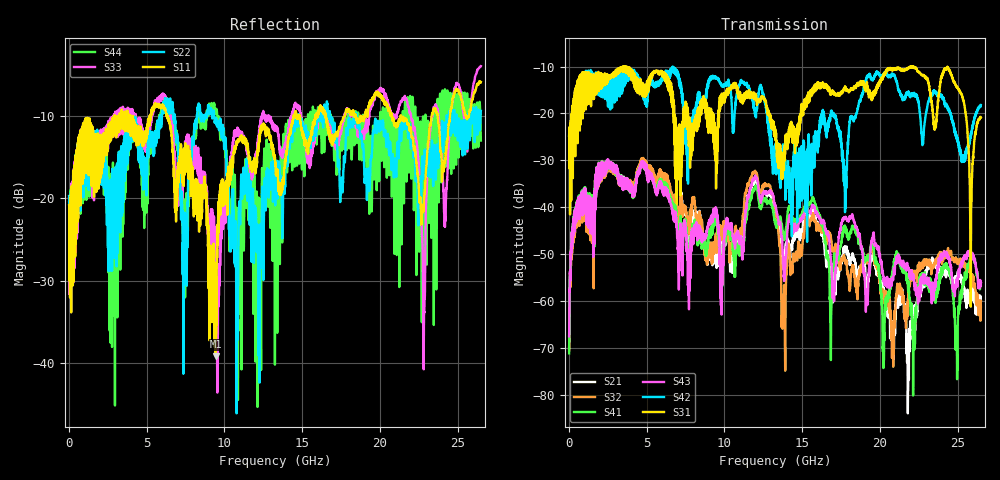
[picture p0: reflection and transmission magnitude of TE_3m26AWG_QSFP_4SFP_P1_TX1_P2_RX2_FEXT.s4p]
!Agilent Technologies,N5222A,MY51421691,A.10.00.00
!Agilent N5222A: A.10.00.00
!Date: Friday, January 30, 2015 12:37:38
!Correction: S11(Full 4 Port(1,2,3,4))
!S12(Full 4 Port(1,2,3,4))
!S13(Full 4 Port(1,2,3,4))
!S14(Full 4 Port(1,2,3,4))
!S21(Full 4 Port(1,2,3,4))
!S22(Full 4 Port(1,2,3,4))
!S23(Full 4 Port(1,2,3,4))
!S24(Full 4 Port(1,2,3,4))
!S31(Full 4 Port(1,2,3,4))
!S32(Full 4 Port(1,2,3,4))
!S33(Full 4 Port(1,2,3,4))
!S34(Full 4 Port(1,2,3,4))
!S41(Full 4 Port(1,2,3,4))
!S42(Full 4 Port(1,2,3,4))
!S43(Full 4 Port(1,2,3,4))
!S44(Full 4 Port(1,2,3,4))
!S4P File: Measurements: <S11,S12,S13,S14>,
!<S21,S22,S23,S24>,
!<S31,S32,S33,S34>,
!<S41,S42,S43,S44>:
# Hz S  dB  R 50.0
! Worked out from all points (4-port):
!   2650 points, 10 MHz to 26.5 GHz, reference 50 ohm
!   strongest paths, dB at 10 MHz, 6.63 GHz, 13.26 GHz, 19.88 GHz, 26.5 GHz:
!     S31: -24.8, -18.2, -24.4, -13.6, -20.8
!     S42: -24.7, -11.1, -30.3, -11.5, -18.2
!     S43: -67.6, -40.3, -39.5, -48.9, -56.2
!     S41: -71.2, -39.3, -43.2, -52.2, -56.7
!     S32: -70.6, -37.1, -40.2, -53.1, -61.3
!     S21: -70.1, -38.3, -42.2, -53.5, -60.1
!   lowest |S11| = -39.2 dB at 9.43 GHz (marker M1), VSWR 1.02, Z = 50.5 + j0.992 ohm
!   |S11| at or under -10 dB: start of sweep to 2.939 GHz; 6.343 GHz to 14.45 GHz (8.108 GHz wide, 78 % of centre); 21.35 GHz to 23.33 GHz (1.977 GHz wide, 8.85 % of centre)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
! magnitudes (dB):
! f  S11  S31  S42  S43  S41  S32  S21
! 10 MHz  -20.9  -24.8  -24.7  -67.6  -71.2  -70.6  -70.1
! 2.5 GHz  -12.1  -11.8  -14.3  -31.8  -31.9  -32.4  -32.3
! 9.43 GHz  -39.2  -27.3  -12.1  -40.3  -42.3  -47.1  -49.8
! 10.98 GHz  -13.0  -15.4  -13.7  -47.9  -50.3  -45.9  -47.8
! 14.28 GHz  -11.9  -24.9  -34.4  -43.0  -40.6  -51.7  -48.7
! 22.81 GHz  -21.6  -11.8  -25.1  -56.1  -55.2  -51.9  -54.9
! 26.5 GHz  -5.9  -20.8  -18.2  -56.2  -56.7  -61.3  -60.1
